(* Logix 5000 AddOnInstructionDefinition export AMCI_SV160E2_Absolute_Move; software revision 20.03 *)

ADD_ON_INSTRUCTION AMCI_SV160E2_Absolute_Move   (* revision 1.0, vendor AMCI, ExecuteEnableInFalse *)
// Revision note:
// 8/2019 Version 0 Initial release of SV160E2 Add On Instructions.
// 3/17/20 Version 1 replaced the generic EDS file with a more complete V1.6 EDS file.
VAR_INPUT
   Status_Word_0 : INT; {required}
        .0   // Set when the SV160E2 is moving CW
        .1   // Set when SV160E2 is moving CCW
        .7   // SV160E2 Move Complete bit
        .11   // Set when there is an input error
        .12   // set when there is a command error
        .13   // set when there is a configuration error
   Status_Word_1 : INT; {required}
        .15   // Set when SV160E2 is enabled
   Type_0_for_standard_1_for_indexed : BOOL;
   Target_Position : DINT; {required}
   Programmed_Speed : DINT; {required}
   Acceleration : INT; {required}
   Deceleration : INT; {required}
   Maximum_Move_Torque : INT;
END_VAR
VAR_IN_OUT
   AMCI_SV160E2_output_data : _000A:SV160E2_9125ACD4:O:0; {required}
END_VAR
VAR_OUTPUT
   EN : BOOL; {access Read Only, visible}   // AOI EN bit
   ER : BOOL; {access Read Only, visible}   // AOI ER bit
END_VAR
VAR
   command_data_block : INT[10];
        [0]   // Command Word 0
        [1]   // Command Word 1
        [2]   // Upper Target Position
        [3]   // Lower Target Position
        [4]   // Upper Programmed Speed
        [5]   // Lower Programmed Speed
END_VAR

ROUTINE EnableInFalse   (* ladder *)
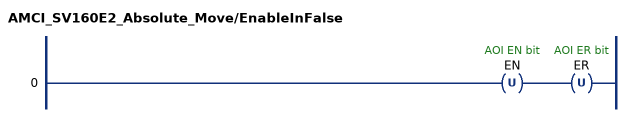
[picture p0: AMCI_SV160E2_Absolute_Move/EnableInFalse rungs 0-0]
   0: OTU(EN)OTU(ER);
END_ROUTINE

ROUTINE Logic   (* ladder *)
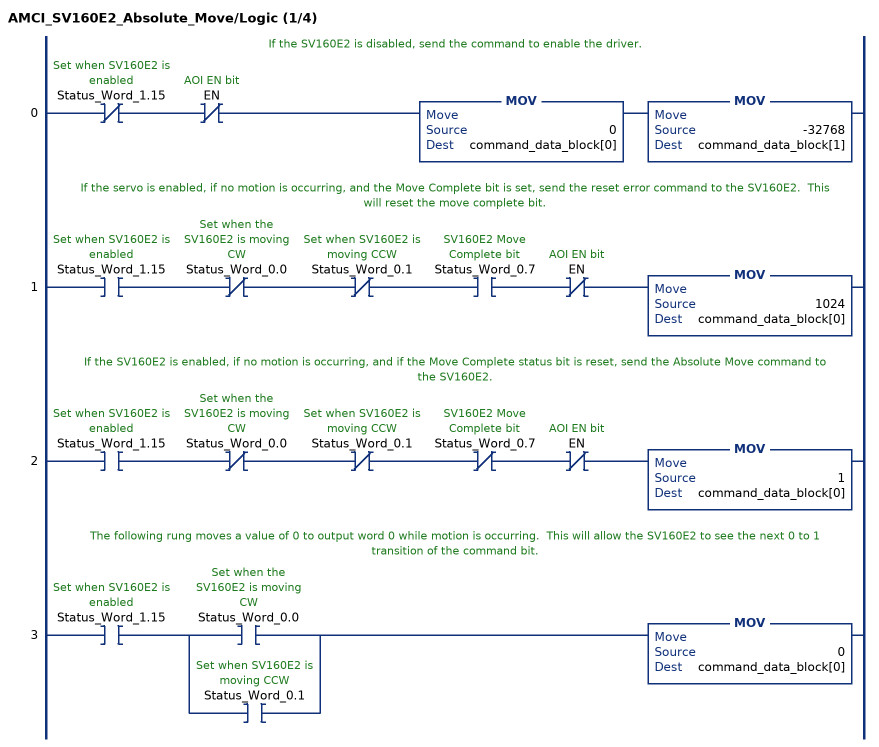
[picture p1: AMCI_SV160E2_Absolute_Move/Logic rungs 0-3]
   // If the SV160E2 is disabled, send the command to enable the driver.
   0: XIO(Status_Word_1.15)XIO(EN)MOV(0,command_data_block[0])MOV(-32768,command_data_block[1]);
   // If the servo is enabled, if no motion is occurring, and the Move Complete bit is set, send the reset error command to the SV160E2.  This will reset the move complete bit.
   1: XIC(Status_Word_1.15)XIO(Status_Word_0.0)XIO(Status_Word_0.1)XIC(Status_Word_0.7)XIO(EN)MOV(1024,command_data_block[0]);
   // If the SV160E2 is enabled, if no motion is occurring, and if the Move Complete status bit is reset, send the Absolute Move command to the SV160E2.
   2: XIC(Status_Word_1.15)XIO(Status_Word_0.0)XIO(Status_Word_0.1)XIO(Status_Word_0.7)XIO(EN)MOV(1,command_data_block[0]);
   // The following rung moves a value of 0 to output word 0 while motion is occurring.  This will allow the SV160E2 to see the next 0 to 1 transition of the command bit.
   3: XIC(Status_Word_1.15)[XIC(Status_Word_0.0) ,XIC(Status_Word_0.1) ]MOV(0,command_data_block[0]);
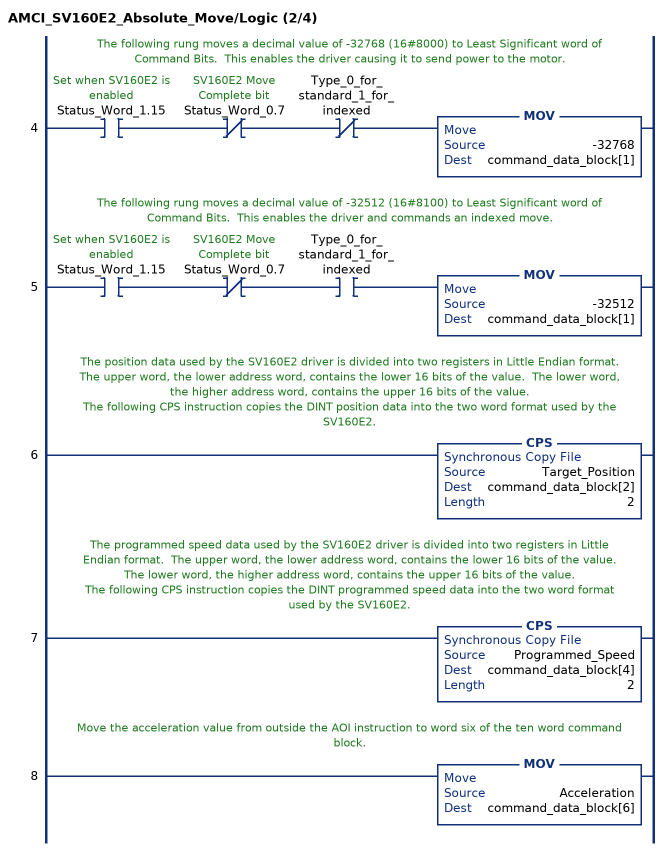
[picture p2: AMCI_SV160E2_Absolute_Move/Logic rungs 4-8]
   // The following rung moves a decimal value of -32768 (16#8000) to Least Significant word of Command Bits.  This enables the driver causing it to send power to the motor.
   4: XIC(Status_Word_1.15)XIO(Status_Word_0.7)XIO(Type_0_for_standard_1_for_indexed)MOV(-32768,command_data_block[1]);
   // The following rung moves a decimal value of -32512 (16#8100) to Least Significant word of Command Bits.  This enables the driver and commands an indexed move.
   5: XIC(Status_Word_1.15)XIO(Status_Word_0.7)XIC(Type_0_for_standard_1_for_indexed)MOV(-32512,command_data_block[1]);
   // The position data used by the SV160E2 driver is divided into two registers in Little Endian format.  The upper word, the lower address word, contains the lower 16 bits of the value.  The lower word, the higher address word, contains the upper 16 bits of the value.
   // The following CPS instruction copies the DINT position data into the two word format used by the SV160E2.
   6: CPS(Target_Position,command_data_block[2],2);
   // The programmed speed data used by the SV160E2 driver is divided into two registers in Little Endian format.  The upper word, the lower address word, contains the lower 16 bits of the value.  The lower word, the higher address word, contains the upper 16 bits of the value.
   // The following CPS instruction copies the DINT programmed speed data into the two word format used by the SV160E2.
   7: CPS(Programmed_Speed,command_data_block[4],2);
   // Move the acceleration value from outside the AOI instruction to word six of the ten word command block.
   8: MOV(Acceleration,command_data_block[6]);
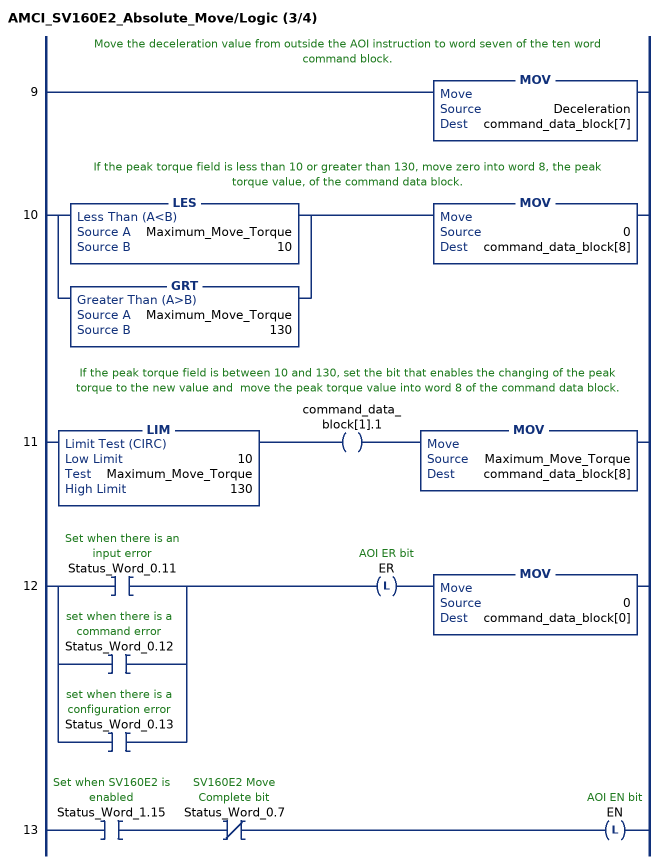
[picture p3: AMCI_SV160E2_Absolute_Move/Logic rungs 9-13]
   // Move the deceleration value from outside the AOI instruction to word seven of the ten word command block.
   9: MOV(Deceleration,command_data_block[7]);
   // If the peak torque field is less than 10 or greater than 130, move zero into word 8, the peak torque value, of the command data block.
   10: [LES(Maximum_Move_Torque,10) ,GRT(Maximum_Move_Torque,130) ]MOV(0,command_data_block[8]);
   // If the peak torque field is between 10 and 130, set the bit that enables the changing of the peak torque to the new value and  move the peak torque value into word 8 of the command data block.
   11: LIM(10,Maximum_Move_Torque,130)OTE(command_data_block[1].1)MOV(Maximum_Move_Torque,command_data_block[8]);
   12: [XIC(Status_Word_0.11) ,XIC(Status_Word_0.12) ,XIC(Status_Word_0.13) ]OTL(ER)MOV(0,command_data_block[0]);
   13: XIC(Status_Word_1.15)XIO(Status_Word_0.7)OTL(EN);
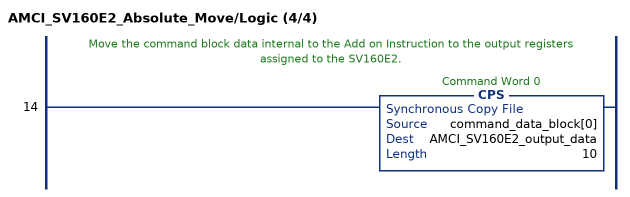
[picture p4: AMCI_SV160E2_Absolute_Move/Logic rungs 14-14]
   // Move the command block data internal to the Add on Instruction to the output registers assigned to the SV160E2.
   14: CPS(command_data_block[0],AMCI_SV160E2_output_data,10);
END_ROUTINE
END_ADD_ON_INSTRUCTION
